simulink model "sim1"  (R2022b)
settings: Solver=VariableStepAuto  StartTime=0.0  StopTime=10.0  FixedStep=0.01  MaxStep=0.05  RelTol=1e-3
InitFcn:
  | a=[-2 1;0 -3];
  | b=[0 1]';
  | c=[1 0];
  | d=0;
libraries: slpidlib x1

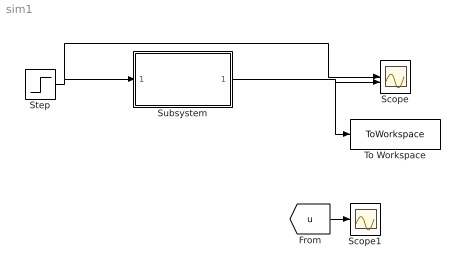
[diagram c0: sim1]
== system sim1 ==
  Scope : Scope  NumInputPorts=2
  Scope1 : Scope
  Step : Step  Time=0  SampleTime=0
  Subsystem : Subsystem
  To Workspace : ToWorkspace  VariableName=sim1  SaveFormat=Structure With Time  SampleTime=-1
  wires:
  Step/1 -> Subsystem/1(In1), Scope/1
  Subsystem/1(Out1) -> To Workspace/1, Scope/2
  [u] -> Scope1/1

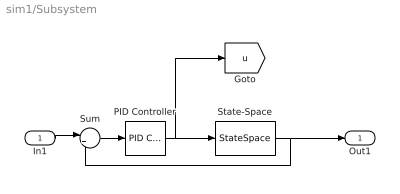
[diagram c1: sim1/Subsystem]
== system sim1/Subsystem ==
  In1 : Inport
  PID Controller : slpidlib/PID Controller  Controller=PID  Form=Ideal  TimeDomain=Continuous-time  UseExternalTs=off  SampleTime=-1  IntegratorMethod=Forward Euler  FilterMethod=Forward Euler  ControllerParametersSource=internal  P=3.60581133071984  I=2.28041202435734  UseKiTs=off  D=0  N=100  UseFilter=on  TunerSelectOption=Transfer Function Based (PID Tuner App)  InitialConditionSource=internal  InitialConditionForIntegrator=0  InitialConditionForFilter=0  DifferentiatorICPrevScaledInput=0  ExternalReset=none  TrackingMode=off  Kt=1  LimitOutput=off  SatLimitsSource=internal  UpperSaturationLimit=inf  LowerSaturationLimit=-inf  LinearizeAsGain=on  AntiWindupMode=none  Kb=1  LimitIntegrator=off  UpperIntegratorSaturationLimit=inf  LowerIntegratorSaturationLimit=-inf  POutMin=[]  POutMax=[]  IOutMin=[]  IOutMax=[]  DOutMin=[]  DOutMax=[]  NOutMin=[]  NOutMax=[]  SumOutMin=[]  SumOutMax=[]  SaturationOutMin=[]  SaturationOutMax=[]  PParamMin=[]  PParamMax=[]  IParamMin=[]  IParamMax=[]  DParamMin=[]  DParamMax=[]  NParamMin=[]  NParamMax=[]  KbParamMin=[]  KbParamMax=[]  KtParamMin=[]  KtParamMax=[]  KbOutMin=[]  KbOutMax=[]  KtOutMin=[]  KtOutMax=[]  IntegratorOutMin=[]  IntegratorOutMax=[]  FilterOutMin=[]  FilterOutMax=[]  SumI1OutMin=[]  SumI1OutMax=[]  SumI2OutMin=[]  SumI2OutMax=[]  SumI3OutMin=[]  SumI3OutMax=[]  SumI4OutMin=[]  SumI4OutMax=[]  SumDOutMin=[]  SumDOutMax=[]  DifferentiatorOutMin=[]  DifferentiatorOutMax=[]  FilterDiffOutCoefMin=[]  FilterDiffOutCoefMax=[]  ReciprocalOutMin=[]  ReciprocalOutMax=[]  SumDenOutMin=[]  SumDenOutMax=[]  SumNumOutMin=[]  SumNumOutMax=[]  DivideOutMin=[]  DivideOutMax=[]  UdiffTsProdOutMin=[]  UdiffTsProdOutMax=[]  NTsProdOutMin=[]  NTsProdOutMax=[]  UintegralTsProdOutMin=[]  UintegralTsProdOutMax=[]  UngainTsProdOutMin=[]  UngainTsProdOutMax=[]  ClampingZeroOutDataTypeStr=Inherit: Inherit via back propagation  ClampingZeroOutMin=[]  ClampingZeroOutMax=[]  FilterDenConstantOutDataTypeStr=Inherit: Inherit via back propagation  FilterDenConstantOutMin=[]  FilterDenConstantOutMax=[]  PCopyOutDataTypeStr=Inherit: Inherit via back propagation  PCopyOutMin=[]  PCopyOutMax=[]  NCopyOutDataTypeStr=Inherit: Inherit via back propagation  NCopyOutMin=[]  NCopyOutMax=[]  IntegratorContinuousStateAttributes=''  IntegratorStateMustResolveToSignalObject=off  IntegratorRTWStateStorageClass=Auto  FilterContinuousStateAttributes=''  FilterStateMustResolveToSignalObject=off  FilterRTWStateStorageClass=Auto  ParallelPVariant=Passthrough  IdealPVariant=InternalParameters  IVariant=InternalParameters  DVariant=InternalParameters  IntegratorVariant=Continuous  SatVariant=Disabled  AWVariant=Passthrough  PCopyVariant=Disabled  TRVariant=Disabled  FdbkBlocksVariant=Forward  IdealPFdbkVariant=Disabled  SatFdbkVariant=Disabled  DerivativeFilterVariant=ContFilter  NVariant=InternalParameters  NCopyVariant=Disabled  FilterICVariant=InternalICsFilter  IntegratorICVariant=InternalICs  ExternalResetVariant=Disabled  TRSumVariant=Passthrough  SumFdbkVariant=Disabled  SumVariant=Sum_PID  TsampFilterVariant=InternalTs  TsampNgainVariant=Passthrough  TsampIntegralVariant=Passthrough  ExternalSaturationOutDataTypeStr=Inherit: Same as second input
  State-Space : StateSpace  A=a  B=b  C=c  D=d  InitialCondition=0
  Sum : Sum  Inputs=|+-
  Out1 : Outport
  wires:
  In1/1 -> Sum/1
  State-Space/1 -> Out1/1, Sum/2
  Sum/1 -> PID Controller/1
  PID Controller/1 -> [u], State-Space/1
